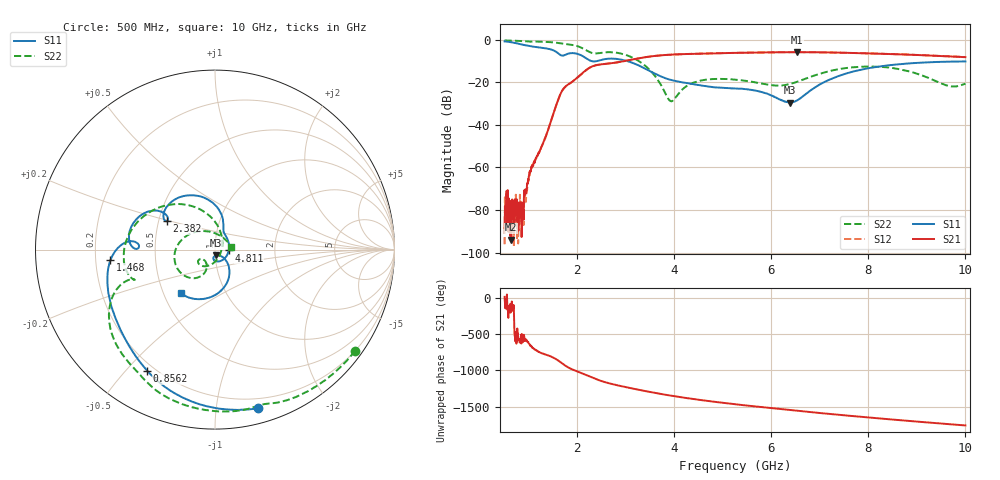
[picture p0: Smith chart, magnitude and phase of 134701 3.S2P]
!  2-Port S-parameters saved by WinCal
! VAR MeasName=S-Parameters (CALIBRATED_DATA) read from VNA (N5242A)
! VAR MeasDate=2013-7-3 16:21:13
! VAR NAME=134701 3
! VAR FILENAME=134701 3.S2P
! VAR DATE=2013-7-3 16:21:13
! VAR PHYS_PORTS=1,2
# Hz S MA R 50
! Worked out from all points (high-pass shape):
!   1601 points, 500 MHz to 10 GHz, reference 50 ohm
!   highest |S21| = -5.83 dB at 6.521 GHz (marker M1); lowest = -94.0 dB at 636.6 MHz (marker M2)
!   |S21| within 3 dB of the highest: 3.238 GHz to end of sweep
!   lowest |S11| = -29.5 dB at 6.39 GHz (marker M3), VSWR 1.07, Z = 50.6 - j3.31 ohm
!   |S11| at or under -10 dB: 2.288 GHz to 2.406 GHz (118.4 MHz wide, 5.04 % of centre); 3.022 GHz to end of sweep
!   |S22| runs from -28.9 to -0.3 dB; largest |S21 - S12| = 0.0035
!   S11 on the Smith chart (normalised r, x): 500 MHz: 0.12, -1.30; 856.2 MHz: 0.17, -0.57; 1.468 GHz: 0.26, -0.05; 2.382 GHz: 0.55, +0.19; 4.811 GHz: 1.17, -0.01; 10 GHz: 0.61, -0.33
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5e8  0.9162 -74.8  3.753e-05 15.1  1.564e-05 -138.9  0.9629 -35.9
6.365625e8  0.8734 -93.2  1.996e-05 -96.6  5.558e-05 100.6  0.9551 -45.6
8.5625e8  0.7737 -119.2  5.66e-05 -137.2  0.0001397 119.4  0.9367 -61.3
9.15625e8  0.7471 -125.1  0.0002403 126.4  0.0002382 159.0  0.9268 -65.6
1.034375e9  0.7042 -135.7  0.0008633 59.9  0.0008514 63.3  0.9026 -73.0
1.467812e9  0.5858 -174.2  0.01358 -92.1  0.01364 -92.5  0.8742 -104.4
1.699375e9  0.4234 177.9  0.06724 170.5  0.06702 170.3  0.809 -121.9
2.085312e9  0.4279 150.3  0.1576 42.5  0.157 42.5  0.6495 -153.4
2.382188e9  0.312 149.6  0.2524 -40.1  0.2514 -40.1  0.4774 -159.4
2.702812e9  0.3604 134.6  0.2812 -105.9  0.2802 -105.9  0.5098 -176.4
3.13625e9  0.2867 99.3  0.3439 -169.6  0.3433 -169.5  0.3812 140.9
3.670625e9  0.1464 71.0  0.4252 121.3  0.4248 121.3  0.1087 74.9
3.937812e9  0.1128 65.1  0.4472 90.7  0.4472 90.7  0.03572 -18.5
4.311875e9  0.09374 46.2  0.4646 52.7  0.465 52.7  0.08948 -106.4
4.810625e9  0.07654 -3.4  0.4805 8.5  0.4802 8.5  0.1193 -133.6
5.25e9  0.07166 -53.0  0.4918 -26.6  0.4918 -26.6  0.1158 -144.7
6.39e9  0.03342 -77.6  0.5098 -107.6  0.5102 -107.7  0.09178 -120.8
6.520625e9  0.03724 -60.2  0.511 -116.4  0.5103 -116.5  0.1017 -116.4
6.835312e9  0.06776 -43.3  0.5091 -137.2  0.5091 -137.1  0.1379 -113.9
7.565625e9  0.1641 -61.1  0.4936 176.9  0.494 177.0  0.2183 -136.0
8.420625e9  0.2513 -89.2  0.4634 126.8  0.4628 126.8  0.2227 -177.8
1e10  0.3089 -128.2  0.3901 40.7  0.392 40.6  0.09285 10.2
